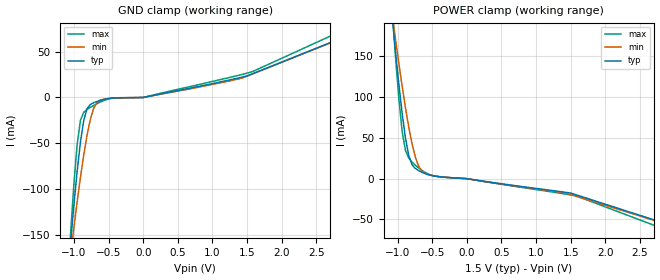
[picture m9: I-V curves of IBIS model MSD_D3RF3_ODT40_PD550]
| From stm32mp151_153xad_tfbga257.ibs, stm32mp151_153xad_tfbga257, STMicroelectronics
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[Model] MSD_D3RF3_ODT40_PD550
Model_type   Input
C_comp 2.313pF   2.272pF   2.391pF
Vinh = 925.000mV
Vinl = 575.000mV
[Temperature Range]   25.000   125.000   -40.000
[Voltage Range]   1.500V   1.425V   1.575V
[GND Clamp Reference]   0.00V   0.00V   0.00V
[POWER Clamp Reference]   1.500V   1.425V   1.575V
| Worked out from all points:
|   GND clamp passes 1 mA (typ) near -0.48 V on its own axis
|   POWER clamp passes 1 mA (typ) near -0.21 V on its own axis
[GND Clamp]
-1.48V    -589.8mA   -457.3mA   -788.8mA
-1.05V    -159.4mA   -171.8mA   -149.6mA
-1.002V   -118mA     -142.3mA   -95.14mA
-954.6mV  -80.6mA    -113.9mA   -51.17mA
-906.8mV  -48.68mA   -87.17mA   -24.84mA
-859.1mV  -24.98mA   -62.62mA   -16.16mA
-763.6mV  -7.616mA   -23.85mA   -10.79mA
-715.9mV  -5.67mA    -11.89mA   -8.7mA
-620.5mV  -3.228mA   -2.934mA   -4.98mA
900nV     14.55nA    13.37nA    17.06nA
1.575V    25.84mA    25.59mA    28.19mA
2.959V    67.83mA    67.3mA     75.92mA
[Power Clamp]
-1.459V   583.2mA    458.9mA    772.5mA
-1.077V   197.8mA    201.5mA    208.1mA
-1.03V    155.3mA    171.1mA    150.1mA
-981.8mV  116.1mA    141.5mA    98.27mA
-934.1mV  80.4mA     113.4mA    58.01mA
-886.4mV  50.05mA    87.11mA    34.74mA
-838.6mV  28.21mA    63.33mA    25.18mA
-790.9mV  17.03mA    42.73mA    20.31mA
-695.5mV  9.8mA      15.23mA    12.99mA
-504.6mV  3.742mA    3.872mA    3.936mA
1.548V    -19.02mA   -20.86mA   -20.65mA
2.98V     -58.14mA   -58.42mA   -66.06mA
